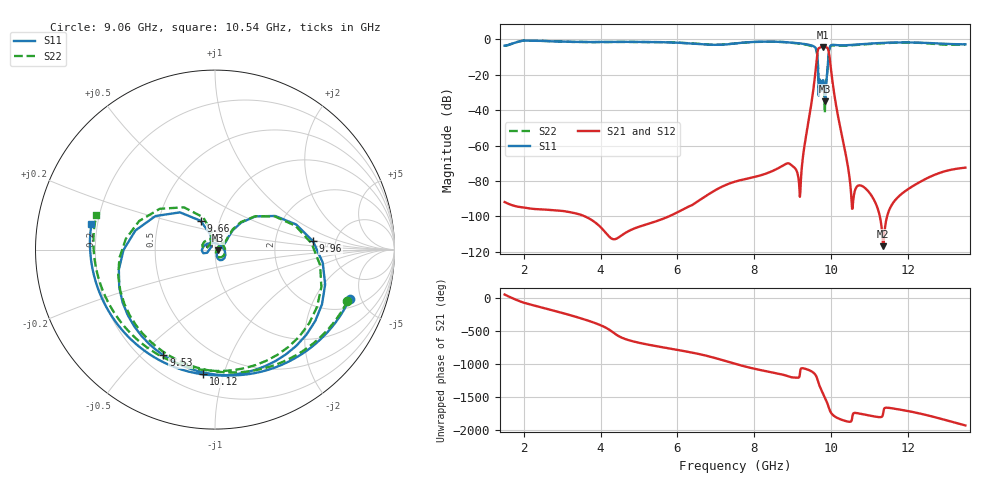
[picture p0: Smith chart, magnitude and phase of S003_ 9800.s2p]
# Hz S DB R 50
! Planar, S50180, , 20.4.1/1
! Date: 14.12.2021 19:01:33
! Data: Format (Calibration Info)
! Freq	S11:dB/Ang(--)	S21:dB/Ang(--)	S12:dB/Ang(--)	S22:dB/Ang(--)
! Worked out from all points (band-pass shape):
!   1201 points, 1.5 GHz to 13.5 GHz, reference 50 ohm
!   highest |S21| = -4.17 dB at 9.78 GHz (marker M1); lowest = -116.8 dB at 11.36 GHz (marker M2)
!   |S21| within 3 dB of the highest: 9.65 GHz to 9.943 GHz (293.2 MHz wide, 2.99 % of centre)
!   lowest |S11| = -35.0 dB at 9.85 GHz (marker M3), VSWR 1.04, Z = 51.8 - j0.453 ohm
!   |S11| at or under -10 dB: 9.646 GHz to 9.933 GHz (286.5 MHz wide, 2.93 % of centre)
!   |S22| runs from -41.5 to -0.5 dB; largest |S21 - S12| = 1.5e-06
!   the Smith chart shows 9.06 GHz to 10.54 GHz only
!   S11 on the Smith chart (normalised r, x): 9.06 GHz: 2.61, -3.98; 9.53 GHz: 0.28, -0.59; 9.66 GHz: 0.81, +0.27; 9.96 GHz: 3.36, +0.45; 10.12 GHz: 0.32, -0.86; 10.54 GHz: 0.18, +0.10
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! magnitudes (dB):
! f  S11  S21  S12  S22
! 1.5 GHz  -3.5  -91.9  -91.9  -3.5
! 3.5 GHz  -1.3  -99.2  -99.2  -1.4
! 5.5 GHz  -1.5  -102.4  -102.4  -1.5
! 7.5 GHz  -2.2  -80.3  -80.3  -2.2
! 8.85 GHz  -1.6  -70.1  -70.1  -1.6
! 9.06 GHz  -1.9  -72.7  -72.7  -2.0
! 9.21 GHz  -2.3  -81.9  -81.9  -2.4
! 9.5 GHz  -3.4  -34.7  -34.7  -3.8
! 9.53 GHz  -3.7  -30.0  -30.0  -4.0
! 9.6 GHz  -4.8  -17.1  -17.1  -5.1
! 9.66 GHz  -14.9  -6.0  -6.0  -14.3
! 9.72 GHz  -23.4  -4.5  -4.5  -22.6
! 9.78 GHz  -23.8  -4.2  -4.2  -24.6
! 9.85 GHz  -35.0  -4.3  -4.3  -32.8
! 9.96 GHz  -5.2  -9.5  -9.5  -5.4
! 10.12 GHz  -3.1  -35.7  -35.7  -3.5
! 10.46 GHz  -3.2  -74.5  -74.5  -3.4
! 10.54 GHz  -3.1  -92.6  -92.6  -3.2
! 11.36 GHz  -1.9  -116.8  -116.8  -2.1
! 11.5 GHz  -1.8  -97.3  -97.3  -2.0
! 12.34 GHz  -1.8  -80.3  -80.3  -1.9
! 13.5 GHz  -2.7  -72.4  -72.4  -2.8
